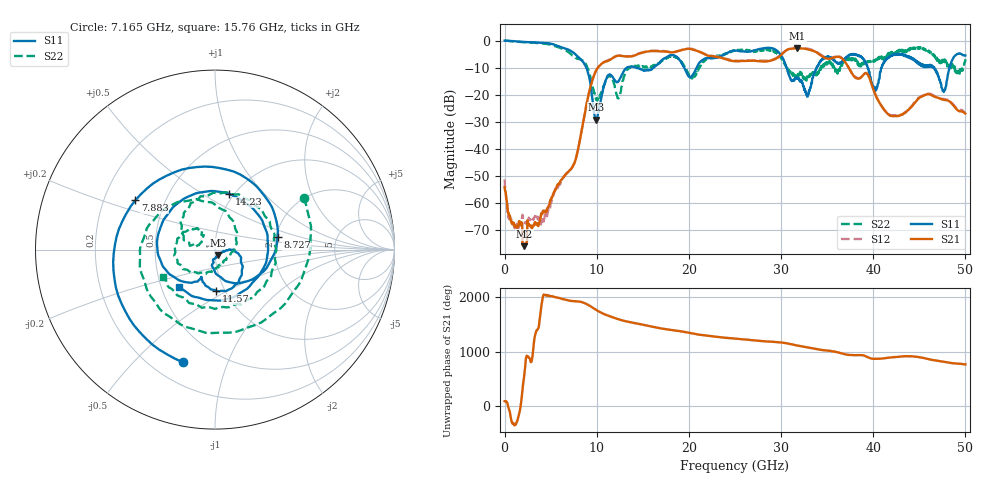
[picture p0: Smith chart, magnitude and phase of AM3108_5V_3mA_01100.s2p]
# Hz S DB R 50.0
!freq dBS11 angS11 dBS21 angS21 dBS12 angS12 dBS22 angS22
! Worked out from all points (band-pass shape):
!   1601 points, 10 MHz to 50 GHz, reference 50 ohm
!   highest |S21| = -2.80 dB at 31.78 GHz (marker M1); lowest = -75.9 dB at 2.166 GHz (marker M2)
!   |S21| within 3 dB of the highest: 13.8 GHz to 22.7 GHz (8.9 GHz wide, 48.8 % of centre); 29.83 GHz to 34.44 GHz (4.612 GHz wide, 14.4 % of centre)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
!   lowest |S11| = -29.1 dB at 9.914 GHz (marker M3), VSWR 1.07, Z = 51.9 - j3.04 ohm
!   |S11| at or under -10 dB: 8.865 GHz to 13.25 GHz (4.384 GHz wide, 39.7 % of centre); 14.28 GHz to 16.17 GHz (1.894 GHz wide, 12.4 % of centre); 30.61 GHz to 33.85 GHz (3.233 GHz wide, 10 % of centre)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
!   |S22| runs from -22.1 to 0.1 dB; largest |S21 - S12| = 0.024
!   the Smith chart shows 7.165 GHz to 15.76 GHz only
!   S11 on the Smith chart (normalised r, x): 7.165 GHz: 0.32, -0.70; 7.883 GHz: 0.34, +0.26; 8.727 GHz: 2.04, +0.32; 11.57 GHz: 0.91, -0.44; 14.23 GHz: 0.95, +0.66; 15.76 GHz: 0.62, -0.28
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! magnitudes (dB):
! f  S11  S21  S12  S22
! 10 MHz  0.0  -54.1  -51.1  0.1
! 1.01 GHz  -0.2  -67.3  -68.1  -0.3
! 2.166 GHz  -0.5  -75.9  -66.5  -0.6
! 4.103 GHz  -0.8  -63.9  -66.2  -1.1
! 7.165 GHz  -3.7  -47.5  -47.6  -4.8
! 7.883 GHz  -5.6  -41.6  -41.6  -6.5
! 8.352 GHz  -7.1  -33.6  -33.6  -7.1
! 8.727 GHz  -9.0  -26.6  -26.5  -8.1
! 9.914 GHz  -29.1  -11.2  -11.1  -21.3
! 11.57 GHz  -12.8  -6.8  -6.6  -13.2
! 12.38 GHz  -14.8  -5.5  -5.5  -21.3
! 14.23 GHz  -9.9  -5.3  -5.2  -9.3
! 15.76 GHz  -10.8  -3.9  -3.7  -9.7
! 16.69 GHz  -8.5  -3.9  -3.6  -8.6
! 25 GHz  -3.7  -7.6  -7.4  -3.7
! 31.78 GHz  -14.1  -2.8  -2.7  -13.5
! 33.35 GHz  -15.5  -3.6  -3.4  -12.7
! 37.88 GHz  -4.9  -13.0  -12.8  -6.4
! 40.22 GHz  -18.6  -19.8  -19.6  -7.6
! 41.69 GHz  -6.1  -27.4  -27.1  -5.2
! 47.66 GHz  -19.0  -21.8  -21.6  -7.6
! 50 GHz  -5.5  -26.9  -26.7  -6.8
